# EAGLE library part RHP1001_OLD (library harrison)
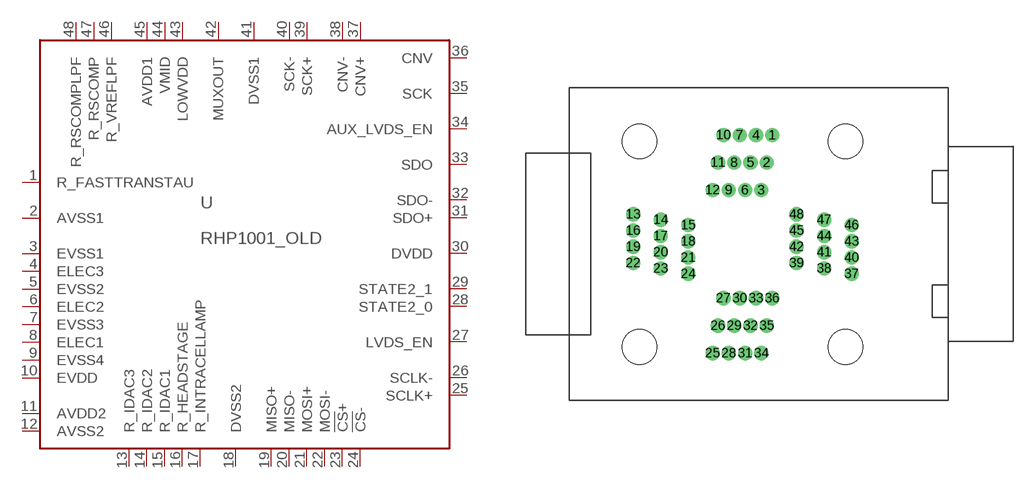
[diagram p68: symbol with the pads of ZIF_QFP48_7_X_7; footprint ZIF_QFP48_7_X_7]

Designator prefix U

## RHP1001_OLD_ZIF_QFP48  [ZIF_QFP48_7_X_7]
1  R_FASTTRANSTAU  pas
2  AVSS1  pwr
3  EVSS1  pwr
4  ELEC3  in
5  EVSS2  pwr
6  ELEC2  in
7  EVSS3  pwr
8  ELEC1  in
9  EVSS4  pwr
10  EVDD  pwr
11  AVDD2  pwr
12  AVSS2  pwr
13  R_IDAC3  pas
14  R_IDAC2  pas
15  R_IDAC1  pas
16  R_HEADSTAGE  pas
17  R_INTRACELLAMP  pas
18  DVSS2  pwr
19  MISO+  out
20  MISO-  out
21  MOSI+  in
22  MOSI-  in
23  !CS!+  in
24  !CS!-  in
25  SCLK+  in
26  SCLK-  in
27  LVDS_EN  in
28  STATE2_0  out
29  STATE2_1  out
30  DVDD  pwr
31  SDO+  out
32  SDO-  out
33  SDO  in
34  AUX_LVDS_EN  in
35  SCK  out
36  CNV  out
37  CNV+  in
38  CNV-  in
39  SCK+  in
40  SCK-  in
41  DVSS1  pwr
42  MUXOUT  out
43  LOWVDD  pwr
44  VMID  pwr
45  AVDD1  pwr
46  R_VREFLPF  pas
47  R_RSCOMP  pas
48  R_RSCOMPLPF  pas

## Footprint ZIF_QFP48_7_X_7 (pad centres in mm)
drill 0.8 pad 1.27: 1 2.75,10.08; 2 2.25,7.54; 3 1.75,5; 4 1.25,10.08; 5 0.75,7.54; 6 0.25,5; 7 -0.25,10.08; 8 -0.75,7.54; 9 -1.25,5; 10 -1.75,10.08; 11 -2.25,7.54; 12 -2.75,5; 13 -10.08,2.75; 14 -7.54,2.25; 15 -5,1.75; 16 -10.08,1.25; 17 -7.54,0.75; 18 -5,0.25; 19 -10.08,-0.25; 20 -7.54,-0.75; 21 -5,-1.25; 22 -10.08,-1.75; 23 -7.54,-2.25; 24 -5,-2.75; 25 -2.75,-10.08; 26 -2.25,-7.54; 27 -1.75,-5; 28 -1.25,-10.08; 29 -0.75,-7.54; 30 -0.25,-5; 31 0.25,-10.08; 32 0.75,-7.54; 33 1.25,-5; 34 1.75,-10.08; 35 2.25,-7.54; 36 2.75,-5; 37 10.08,-2.75; 38 7.54,-2.25; 39 5,-1.75; 40 10.08,-1.25; 41 7.54,-0.75; 42 5,-0.25; 43 10.08,0.25; 44 7.54,0.75; 45 5,1.25; 46 10.08,1.75; 47 7.54,2.25; 48 5,2.75
hole 3.2 at 9.5,9.5
hole 3.2 at -9.5,9.5
hole 3.2 at -9.5,-9.5
hole 3.2 at 9.5,-9.5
